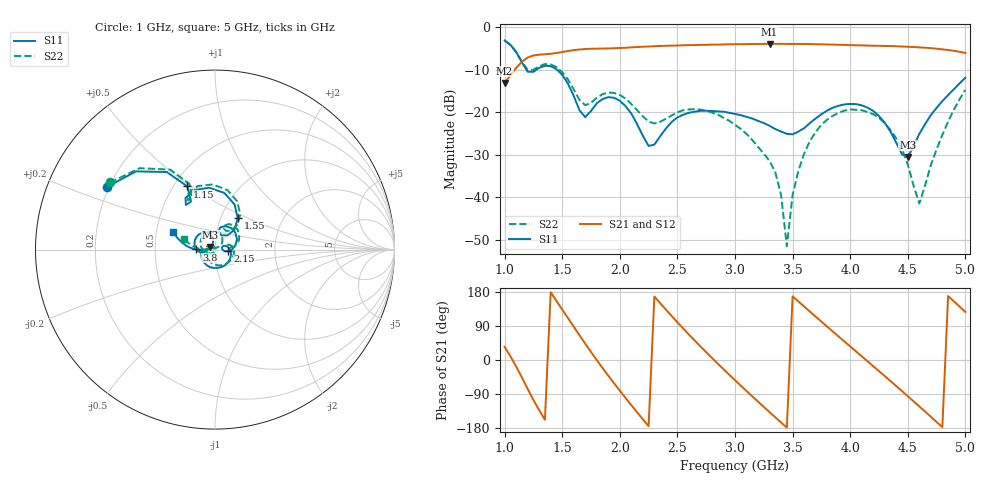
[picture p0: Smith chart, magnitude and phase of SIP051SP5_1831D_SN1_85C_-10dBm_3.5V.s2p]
# GHz  S  dB  R  50
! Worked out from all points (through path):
!   81 points, 1 GHz to 5 GHz, reference 50 ohm
!   highest |S21| = -3.95 dB at 3.3 GHz (marker M1); lowest = -13.1 dB at 1 GHz (marker M2)
!   lowest |S11| = -30.5 dB at 4.5 GHz (marker M3), VSWR 1.06, Z = 47.5 + j1.45 ohm
!   |S11| at or under -10 dB: 1.189 GHz to 1.278 GHz (89.54 MHz wide, 7.26 % of centre); 1.454 GHz to end of sweep
!   |S22| runs from -51.5 to -3.2 dB; largest |S21 - S12| = 0.0023
!   S11 on the Smith chart (normalised r, x): 1 GHz: 0.19, +0.26; 1.15 GHz: 0.59, +0.48; 1.55 GHz: 1.20, +0.44; 2.15 GHz: 1.15, -0.02; 3.8 GHz: 0.81, +0.00; 5 GHz: 0.61, +0.13
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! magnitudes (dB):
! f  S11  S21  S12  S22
! 1 GHz  -3.2  -13.1  -13.1  -3.2
! 1.15 GHz  -8.3  -8.1  -8.1  -8.1
! 1.55 GHz  -13.3  -5.6  -5.6  -12.3
! 1.7 GHz  -21.2  -5.2  -5.2  -18.4
! 1.95 GHz  -16.6  -5.0  -5.0  -15.5
! 2.15 GHz  -22.8  -4.7  -4.7  -19.5
! 2.25 GHz  -27.9  -4.6  -4.6  -22.2
! 2.35 GHz  -25.7  -4.5  -4.4  -22.3
! 2.6 GHz  -20.2  -4.3  -4.2  -19.4
! 3 GHz  -20.4  -4.0  -4.0  -23.0
! 3.3 GHz  -23.2  -4.0  -4.0  -31.5
! 3.4 GHz  -24.6  -4.0  -3.9  -39.5
! 3.45 GHz  -25.1  -4.0  -3.9  -51.5
! 3.5 GHz  -25.2  -4.0  -4.0  -39.5
! 3.55 GHz  -24.6  -4.0  -4.0  -33.8
! 3.7 GHz  -21.5  -4.0  -4.0  -24.7
! 3.8 GHz  -19.6  -4.1  -4.1  -21.8
! 4.1 GHz  -18.4  -4.3  -4.3  -19.5
! 4.35 GHz  -24.6  -4.5  -4.5  -24.2
! 4.5 GHz  -30.5  -4.6  -4.6  -32.3
! 4.6 GHz  -25.1  -4.8  -4.8  -41.5
! 5 GHz  -11.9  -6.1  -6.1  -14.8
